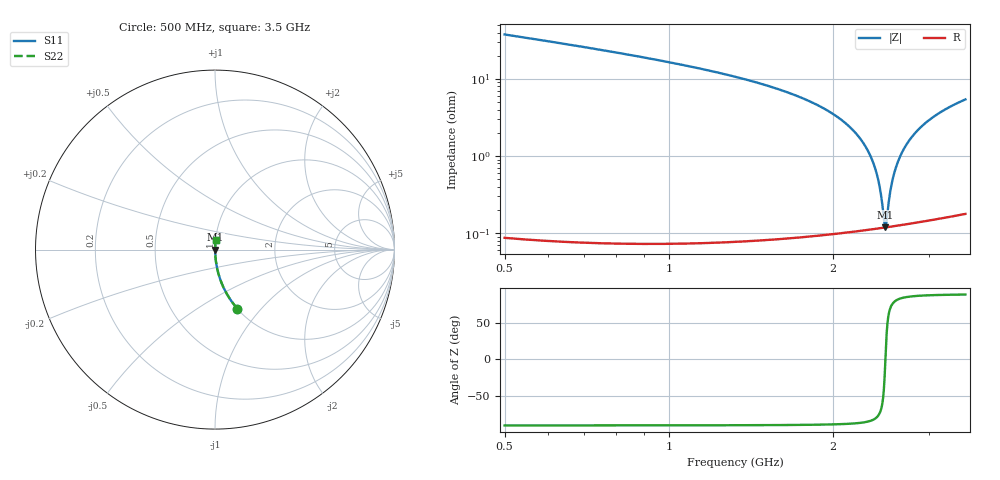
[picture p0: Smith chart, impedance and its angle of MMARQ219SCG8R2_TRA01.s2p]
! MMARQ219SCG8R2_TRA01  S-PARAMETER MODEL  ( General Type )
! Model Generated by TAIYO YUDEN Corporation (http://www.ty-top.com)
! Version 1.0
! TAIYO YUDEN Control No. 160201
! Copyright(c) 2016 TAIYO YUDEN CO.,LTD. All Rights Reserved.
! Product Description (link to TY-COMPAS)
! https://ds.yuden.co.jp/TYCOMPAS/or/detail?pn=MMARQ219SCG8R2CTRA01&u=M
! Products Name : Multilayer Ceramic Capacitors
! Characteristics :
!  Capacitance : 8.2 pF , Rated Voltage : 250V , TCC : CG / C0G
!  Case Size : 2.0 x 1.25 / 0.079 x 0.049 [mm/inch] , Thickness : 0.85 / 0.033 [mm/inch]
!  (Conditions: Temperature = 25 degC , DC Bias Current/Voltage = 0A / 0V)
! External Node Assignments :
!  1  o---| |---o  2
! GND o---------o GND
! Frequency Range : 500MHz  -  3500MHz  [ 401 STEP ]
# MHz S RI R 50
! Freq[MHz].  S11 Real  S11 Imag  S21 Real  S21 Imag  S12 Real  S12 Imag  S22 Real  S22 Imag
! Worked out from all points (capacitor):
!   401 points, 500 MHz to 3.5 GHz, reference 50 ohm
!   read as one part in series: C = 8.1 pF near 515 MHz
!   lowest |Z| = 119 mohm at 2.495 GHz (marker M1)
!   series resonance near 2.497 GHz, so ESL is about 500 pH
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500  0.1252 -0.3299  0.8748 0.3299  0.8748 0.3299  0.1252 -0.3299
1002.5  0.027 -0.1599  0.973 0.1599  0.973 0.1599  0.027 -0.1599
1505  0.00766 -0.0824  0.9923 0.0824  0.9923 0.0824  0.00766 -0.0824
1790  0.00373 -0.0531  0.9963 0.0531  0.9963 0.0531  0.00373 -0.0531
2000  0.0022 -0.0351  0.9978 0.0351  0.9978 0.0351  0.0022 -0.0351
2202.5  0.00144 -0.0197  0.9986 0.0197  0.9986 0.0197  0.00144 -0.0197
2337.5  0.00121 -0.0104  0.9988 0.0104  0.9988 0.0104  0.00121 -0.0104
2382.5  0.00118 -0.00735  0.9988 0.00735  0.9988 0.00735  0.00118 -0.00735
2420  0.00117 -0.0049  0.9988 0.0049  0.9988 0.0049  0.00117 -0.0049
2450  0.00117 -0.00296  0.9988 0.00296  0.9988 0.00296  0.00117 -0.00296
2480  0.00118 -0.00105  0.9988 0.00105  0.9988 0.00105  0.00118 -0.00105
2495  0.00118 -0.000101  0.9988 0.000101  0.9988 0.000101  0.00118 -0.000101
2502.5  0.00119 0.00037  0.9988 -0.00037  0.9988 -0.00037  0.00119 0.00037
2547.5  0.00122 0.00317  0.9988 -0.00317  0.9988 -0.00317  0.00122 0.00317
2570  0.00124 0.00455  0.9988 -0.00455  0.9988 -0.00455  0.00124 0.00455
2607.5  0.00128 0.00683  0.9987 -0.00683  0.9987 -0.00683  0.00128 0.00683
2652.5  0.00135 0.00952  0.9986 -0.00952  0.9986 -0.00952  0.00135 0.00952
2712.5  0.00146 0.013  0.9985 -0.013  0.9985 -0.013  0.00146 0.013
2795  0.00165 0.0178  0.9983 -0.0178  0.9983 -0.0178  0.00165 0.0178
3005  0.00231 0.0292  0.9977 -0.0292  0.9977 -0.0292  0.00231 0.0292
3230  0.00326 0.0408  0.9967 -0.0408  0.9967 -0.0408  0.00326 0.0408
3500  0.00468 0.0538  0.9953 -0.0538  0.9953 -0.0538  0.00468 0.0538
